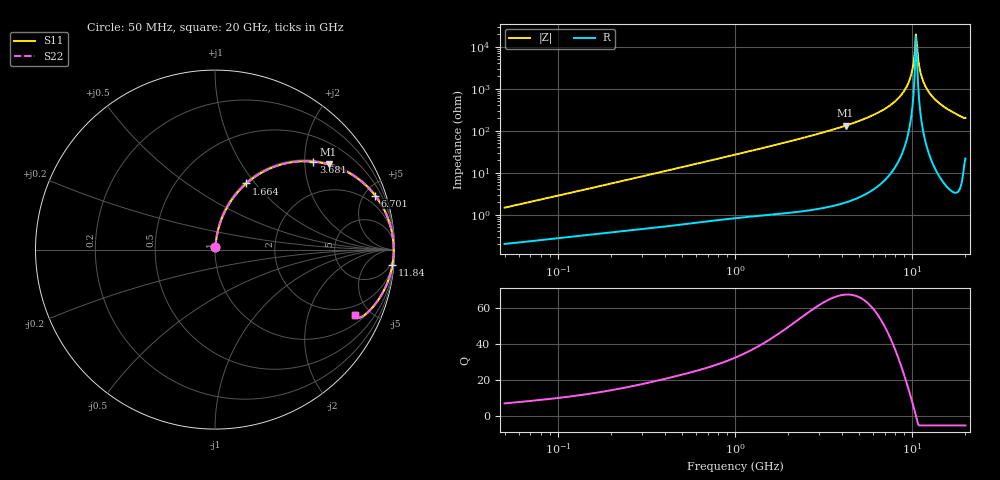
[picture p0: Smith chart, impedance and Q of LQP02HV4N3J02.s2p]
!Murata Part Number: LQP02HV4N3J02
!These Parameters are Measured in Series Mode Connection
!  o--[Z]--o
!Port1  Port2
!  o-------o
!Freq. Start=50[MHz] Stop=20[GHz], 401[Steps]
# Hz S RI R 50
!Freq.(Hz) S11(Real) S11(Imag) S21(Real) S21(Imag) S12(Real) S12(Imag) S22(Real) S22(Imag)
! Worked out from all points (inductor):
!   401 points, 50 MHz to 20 GHz, reference 50 ohm
!   read as one part in series: L = 4.59 nH near 51.52 MHz
!   highest Q = 67.5 at 4.212 GHz (marker M1), where L = 4.98 nH
!   self-resonance near 10.5 GHz
!   S11 on the Smith chart (normalised r, x): 50 MHz: 1.00, +0.03; 1.664 GHz: 1.02, +0.90; 3.681 GHz: 1.03, +2.20; 6.701 GHz: 1.11, +5.91; 11.84 GHz: 2, -24; 20 GHz: 1.43, -4.02
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5e7  0.00222 0.0145  0.9978 -0.0145  0.9978 -0.0145  0.00222 0.0145
1.364002e8  0.00462 0.0378  0.9954 -0.0378  0.9954 -0.0378  0.00462 0.0378
3.721004e8  0.015 0.099  0.985 -0.099  0.985 -0.099  0.015 0.099
1e9  0.0738 0.2465  0.9262 -0.2465  0.9262 -0.2465  0.0738 0.2465
1.664083e9  0.1745 0.3684  0.8255 -0.3684  0.8255 -0.3684  0.1745 0.3684
2.728004e9  0.3741 0.4755  0.6259 -0.4755  0.6259 -0.4755  0.3741 0.4755
3.680849e9  0.5479 0.4902  0.4521 -0.4902  0.4521 -0.4902  0.5479 0.4902
4.212059e9  0.6326 0.4747  0.3674 -0.4747  0.3674 -0.4747  0.6326 0.4747
6.701223e9  0.8927 0.3003  0.1073 -0.3003  0.1073 -0.3003  0.8927 0.3003
7.442007e9  0.9335 0.2382  0.0665 -0.2382  0.0665 -0.2382  0.9335 0.2382
8.516016e9  0.9717 0.1501  0.0283 -0.1501  0.0283 -0.1501  0.9717 0.1501
9.316812e9  0.9874 0.0878  0.0126 -0.0878  0.0126 -0.0878  0.9874 0.0878
9.892087e9  0.9933 0.0454  0.00669 -0.0454  0.00669 -0.0454  0.9933 0.0454
1.034674e10  0.9953 0.0132  0.00467 -0.0132  0.00467 -0.0132  0.9953 0.0132
1.050288e10  0.9955 0.00248  0.00446 -0.00248  0.00446 -0.00248  0.9955 0.00248
1.082228e10  0.9953 -0.019  0.00475 0.019  0.00475 0.019  0.9953 -0.019
1.115139e10  0.994 -0.0405  0.00597 0.0405  0.00597 0.0405  0.994 -0.0405
1.183995e10  0.9888 -0.0832  0.0112 0.0832  0.0112 0.0832  0.9888 -0.0832
1.276073e10  0.9771 -0.1357  0.0229 0.1357  0.0229 0.1357  0.9771 -0.1357
1.438523e10  0.9465 -0.2164  0.0535 0.2164  0.0535 0.2164  0.9465 -0.2164
1.721783e10  0.8743 -0.3252  0.1257 0.3252  0.1257 0.3252  0.8743 -0.3252
2e10  0.7793 -0.3641  0.2207 0.3641  0.2207 0.3641  0.7793 -0.3641
